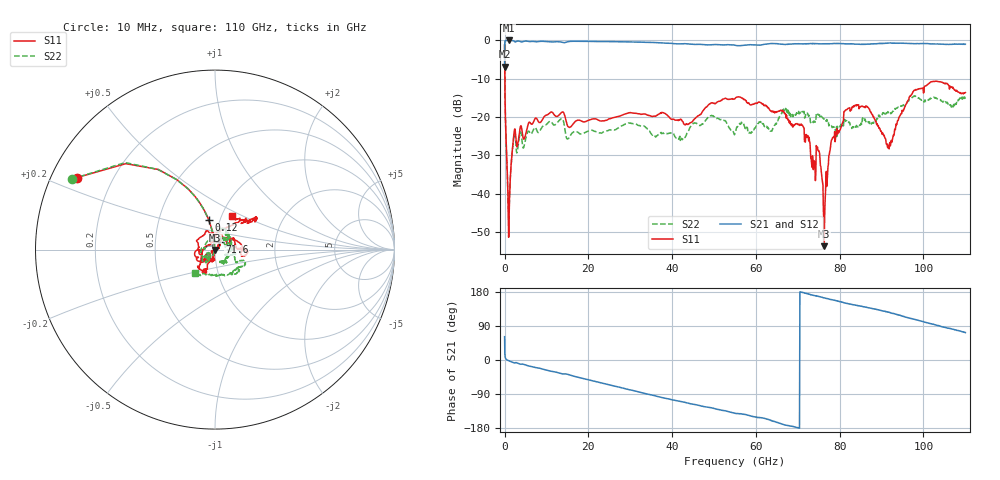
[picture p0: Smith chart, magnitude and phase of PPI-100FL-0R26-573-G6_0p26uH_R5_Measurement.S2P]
! Data measured by Modelithics Inc.  support@modelithics.com  813-866-6335  Tampa FL USA June 2025
! PPI-100FL-0R26-573-G6_0p26uH measured on 5-mil thick RO3003G2 board, mounted in 2-port shunt configuration on a 50-ohm transmission line
# GHz S RI R 50.0
!freq ReS11 ImS11 ReS21 ImS21 ReS12 ImS12 ReS22 ImS22
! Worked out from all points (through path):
!   1207 points, 10 MHz to 110 GHz, reference 50 ohm
!   highest |S21| = -0.03 dB at 979.6 MHz (marker M1); lowest = -6.9 dB at 10 MHz (marker M2)
!   group delay of S21, straight-line fit = 7.18 ps
!   lowest |S11| = -53.7 dB at 76.3 GHz (marker M3), VSWR 1.00, Z = 50.1 - j0.153 ohm
!   |S11| at or under -10 dB: 60.44 MHz to end of sweep
!   |S22| runs from -48.4 to -1.0 dB; largest |S21 - S12| = 0.077
!   S11 on the Smith chart (normalised r, x): 10 MHz: 0.07, +0.24; 120 MHz: 0.89, +0.30; 71.6 GHz: 1.05, +0.09; 110 GHz: 1.12, +0.44
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0.01  -0.7701 0.4008  0.2157 0.3972  0.2158 0.3971  -0.7989 0.3927
0.12  -0.0343 0.1634  0.9654 0.1592  0.9654 0.1591  -0.035 0.1637
0.2  -0.0143 0.0986  0.9854 0.0916  0.9853 0.0916  -0.0148 0.0988
0.9796215  -0.00267 0.000448  0.9961 -0.0329  0.9959 -0.0327  -0.00376 0.000571
2.241776  -0.0263 -0.0554  0.9684 -0.1289  0.9683 -0.1289  -0.0315 -0.0476
6.028239  -0.058 -0.0624  0.9245 -0.2687  0.9245 -0.2692  -0.0399 -0.0481
13.40699  -0.1037 -0.0425  0.7741 -0.5545  0.7733 -0.5557  -0.0596 -0.0731
18.35852  -0.0877 -0.0121  0.6523 -0.715  0.6522 -0.7151  -0.0331 -0.0504
36.7083  -0.0547 0.0938  -0.1099 -0.9244  -0.1132 -0.9239  -0.0588 0.00345
43.50451  0.0386 0.0712  -0.3557 -0.8272  -0.3565 -0.8271  0.024 0.0567
49.23275  0.1506 0.0209  -0.5133 -0.7098  -0.5117 -0.7109  0.103 0.011
55.05808  0.176 -0.00387  -0.6692 -0.544  -0.6648 -0.5494  0.0597 0.0226
71.6  0.0249 0.041  -0.9002 0.051  -0.9044 0.0203  0.069 0.0681
73.4  0.0187 0.0119  -0.8989 0.1404  -0.9008 0.0853  0.0665 0.0524
75  0.0218 0.0293  -0.8809 0.1948  -0.8882 0.1661  0.0885 0.0601
76.3  0.0014 -0.00153  -0.866 0.2512  -0.8801 0.2083  0.093 0.0149
78  -0.00949 -0.0486  -0.8458 0.3176  -0.8634 0.2662  0.075 -0.0182
81.6  -0.0597 -0.1096  -0.7738 0.4556  -0.8017 0.3944  0.0455 -0.0771
86.8  -0.0896 -0.0985  -0.663 0.5994  -0.6916 0.5625  0.0587 -0.0643
91.7  -0.0287 0.0282  -0.546 0.7406  -0.5497 0.7416  0.1096 -0.0312
98  0.154 0.1633  -0.2632 0.8669  -0.2948 0.8555  0.1642 -0.0859
110  0.093 0.1869  0.2709 0.8492  0.2548 0.8574  -0.1133 -0.1301
